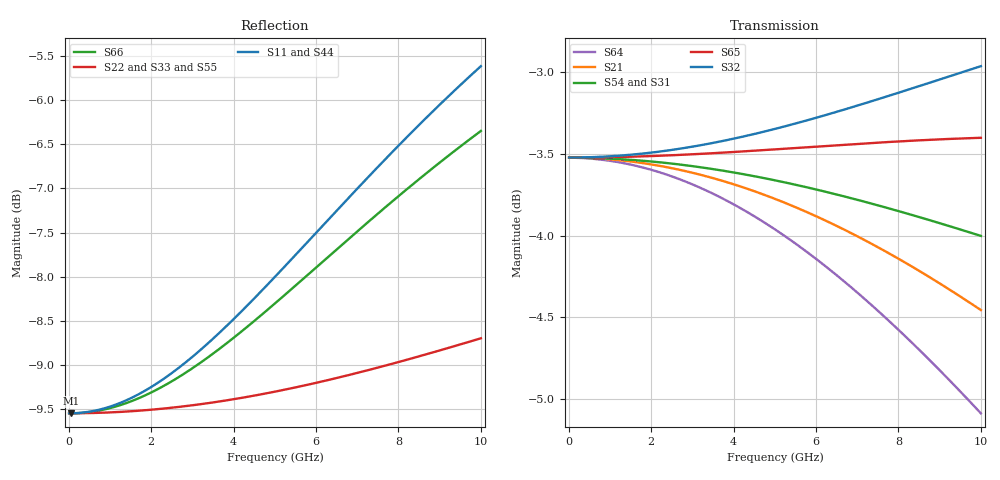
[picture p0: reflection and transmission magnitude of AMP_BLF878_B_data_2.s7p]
! Created Wed Mar 10 14:49:29 2010
# ghz S ma R 50
! 7 Port Network Data from SP1.SP block
! freq  magS11  angS11  magS12  angS12  magS13  angS13  magS14  angS14
!  magS15  angS15  magS16  angS16  magS17  angS17
!  magS21  angS21
!  magS22  angS22  magS23  angS23  magS24  angS24  magS25  angS25
!  magS26  angS26  magS27  angS27
!  magS31  angS31  magS32  angS32
!  magS33  angS33  magS34  angS34  magS35  angS35  magS36  angS36
!  magS37  angS37
!  magS41  angS41  magS42  angS42  magS43  angS43
!  magS44  angS44  magS45  angS45  magS46  angS46  magS47  angS47
!  magS51  angS51  magS52  angS52  magS53  angS53  magS54  angS54
!  magS55  angS55  magS56  angS56  magS57  angS57
!  magS61  angS61
!  magS62  angS62  magS63  angS63  magS64  angS64  magS65  angS65
!  magS66  angS66  magS67  angS67
!  magS71  angS71  magS72  angS72
!  magS73  angS73  magS74  angS74  magS75  angS75  magS76  angS76
!  magS77  angS77
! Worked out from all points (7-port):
!   1000 points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, 10 MHz to 10 GHz, reference 50 ohm
!   strongest paths, dB at 10 MHz, 2.51 GHz, 5.01 GHz, 7.51 GHz, 10 GHz:
!     S32: -3.5, -3.5, -3.3, -3.2, -3.0
!     S65: -3.5, -3.5, -3.5, -3.4, -3.4
!     S54: -3.5, -3.6, -3.7, -3.8, -4.0
!     S31: -3.5, -3.6, -3.8, -4.0, -4.4
!     S21: -3.5, -3.6, -3.8, -4.1, -4.5
!     S64: -3.5, -3.6, -4.0, -4.5, -5.1
!   lowest |S11| = -9.5 dB at 50 MHz (marker M1), VSWR 2.00, Z = 25 + j0.179 ohm
!   |S11| at or under -10 dB: nowhere
